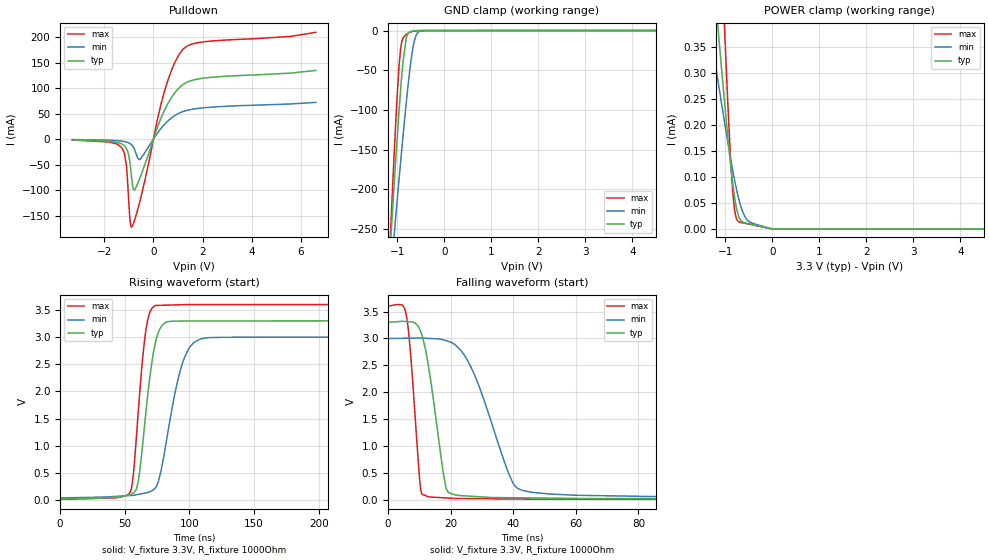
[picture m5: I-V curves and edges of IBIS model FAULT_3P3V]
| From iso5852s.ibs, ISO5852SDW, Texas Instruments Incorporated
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|   Model FAULT_3P3V
[Model]   FAULT_3P3V
Model_type   Open_drain
Polarity   Non-Inverting
Vmeas = 1.65
Vref = 3.3
Cref = 5pF
Rref = 1000
|   typ   min   max
|   (nom PVT)   (slow PVT)   (fast PVT)
C_comp   1.287p   1.250p   1.396p
|C_comp (ON state)   1.437p   1.349p   1.599p
|C_comp (OFF state)   1.287p   1.250p   1.396p
| Where   nom PVT is  Nominal Process, 3.3V, 27C
|   Fast PVT is Strong Process, 3.6V, -40C
|   Slow PVT is Weak Process, 3.0V, 150C
[Voltage Range]   3.3   3   3.6
[Temperature Range]   27   150   -40
[Pullup Reference]   3.3   3   3.6
[Pulldown Reference]   0   0   0
[Power Clamp Reference]   3.3   3   3.6
[GND Clamp Reference]   0   0   0
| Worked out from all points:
|   slope of the pulldown table from 0 to 0.495 V, typ, clamps not added: 8.14 ohm
|   GND clamp passes 1 mA (typ) near -0.71 V on its own axis
|   falling waveform, V_fixture 3.3V, R_fixture 1000Ohm: 20-80 % time 4.75ns typ, 10.7ns min, 2.68ns max; typ from 3.3 V to 0.022 V
|   rising waveform, V_fixture 3.3V, R_fixture 1000Ohm: 20-80 % time 9.41ns typ, 14.4ns min, 7.44ns max; typ from 0.022 V to 3.3 V
[Pulldown]
|   Voltage   I(typ)   I(min)   I(max)
-3.3V     -1.49mA    -939.1uA   -1.943mA
-1.28V    -9.81mA    -4.131mA   -17.78mA
-1.102V   -18.36mA   -5.856mA   -51.29mA
-953.7mV  -47.62mA   -8.834mA   -158.5mA
-894.3mV  -73.8mA    -10.96mA   -172.7mA
-765.6mV  -99.93mA   -20.36mA   -158.4mA
-557.7mV  -77.22mA   -40.23mA   -123mA
432.3mV   54.77mA    27.89mA    90.84mA
808.5mV   86.77mA    44.1mA     143.4mA
1.204V    106.9mA    53.93mA    176mA
1.957V    118.8mA    60.84mA    190mA
6.6V      134.5mA    71.8mA     209.1mA
[GND Clamp]
|   Voltage   I(typ)   I(min)   I(max)
-3.3V     -2.497A    -1.9A      -3.341A
-1.181V   -300mA     -335mA     -298.4mA
-1.112V   -233.2mA   -286.6mA   -207.7mA
-1.063V   -186.8mA   -252.4mA   -146mA
-973.5mV  -107.5mA   -192.2mA   -50.73mA
-933.9mV  -75.44mA   -166.1mA   -23.61mA
-884.4mV  -40.68mA   -134.3mA   -9.594mA
-815.1mV  -10.15mA   -92.08mA   -4.858mA
-726mV    -1.338mA   -44.52mA   -2.024mA
-607.2mV  -206.9uA   -6.808mA   -349.7uA
-448.8mV  -78.53uA   -205.6uA   -79.96uA
6.6V      0A         0A         0A
[POWER Clamp]
|   Voltage   I(typ)   I(min)   I(max)
-3.3V     2.757mA    1.599mA    5.915mA
-1.399V   643.8uA    426.6uA    1.267mA
-1.31V    547.9uA    373.6uA    1.056mA
-1.181V   411.3uA    298uA      754.4uA
-1.013V   239.1uA    202.1uA    376.1uA
-924mV    154.4uA    153.7uA    195.7uA
-844.8mV  88.42uA    113.3uA    73.51uA
-785.4mV  50.68uA    85.59uA    27.02uA
-706.2mV  21.72uA    54.52uA    13.49uA
-528mV    10.57uA    16.67uA    9.759uA
-3.3mV    50.08nA    67.76nA    46.55nA
6.6V      0A         0A         0A
[Ramp]
R_load = 1000
|   typ   min   max
dV/dt_r   1.96663/9.37125e-09   1.77589/1.43584e-08   2.1513/7.4139e-09
dV/dt_f   1.9666/4.75373e-09   1.77549/1.06671e-08   2.1513/2.67533e-09
[Falling Waveform]
V_fixture = 3.3V
V_fixture_min = 3V
V_fixture_max = 3.6V
R_fixture = 1000Ohm
C_fixture = 0F
|   Time   V(typ)   V(min)   V(max)
0s        3.3V       3V         3.6V
5.81ns    3.315V     3.005V     3.439V
7.199ns   3.309V     3.006V     2.716V
10.39ns   3.134V     3.008V     216.1mV
12.76ns   2.537V     3.002V     65.16mV
19.15ns   151.3mV    2.949V     38.48mV
26.87ns   70.64mV    2.422V     28.26mV
40.04ns   44.06mV    307mV      21.57mV
44.97ns   40.81mV    154.6mV    19.06mV
299.9ns   22.33mV    40.85mV    14.5mV
[Rising Waveform]
V_fixture = 3.3V
V_fixture_min = 3V
V_fixture_max = 3.6V
R_fixture = 1000Ohm
C_fixture = 0F
|   Time   V(typ)   V(min)   V(max)
0s        22.29mV    40.17mV    14.49mV
54.31ns   101.1mV    85.04mV    151.5mV
56.52ns   128.6mV    89.17mV    456.2mV
60.1ns    308.9mV    104.3mV    1.525V
65.92ns   1.522V     131.1mV    3.061V
73.2ns    2.848V     214.3mV    3.575V
78.94ns   3.222V     649.9mV    3.586V
93.56ns   3.295V     2.441V     3.596V
107.3ns   3.297V     2.954V     3.599V
299.9ns   3.3V       3V         3.6V
